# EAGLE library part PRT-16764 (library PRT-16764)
Headers & Wire Housings Extended GPIO Female Header - 2x20 Pin (13.5mm/9.80mm) Source: Datasheet
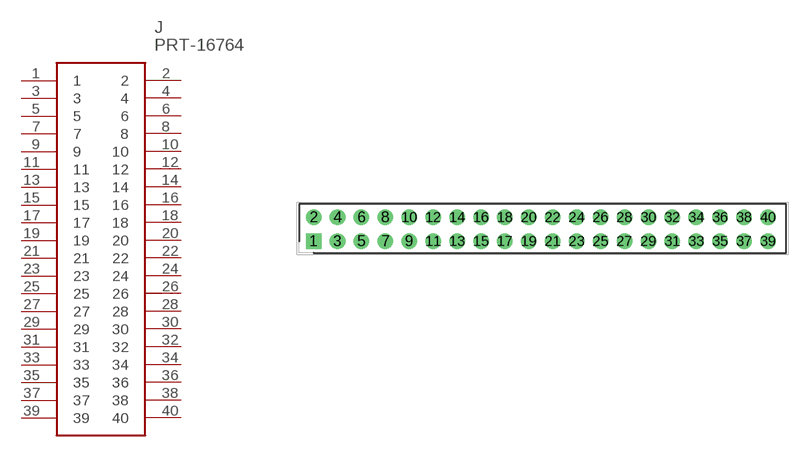
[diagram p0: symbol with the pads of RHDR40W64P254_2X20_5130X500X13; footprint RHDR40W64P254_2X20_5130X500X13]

Designator prefix J

## PRT-16764 (Description: Headers & Wire Housings Extended GPIO Female Header - 2x20 Pin (13.5mm/9.80mm); Height: 13.75mm; Manufacturer_Name: SparkFun; Manufacturer_Part_Number: PRT-16764; Mouser_Part_Number: 474-PRT-16764; Mouser_Price-Stock: https://www.mouser.co.uk/ProductDetail/SparkFun/PRT-16764?qs=W%2FMpXkg%252BdQ4FKwyaXnhaEw%3D%3D)  [RHDR40W64P254_2X20_5130X500X13]
1  1
2  2
3  3
4  4
5  5
6  6
7  7
8  8
9  9
10  10
11  11
12  12
13  13
14  14
15  15
16  16
17  17
18  18
19  19
20  20
21  21
22  22
23  23
24  24
25  25
26  26
27  27
28  28
29  29
30  30
31  31
32  32
33  33
34  34
35  35
36  36
37  37
38  38
39  39
40  40

## Footprint RHDR40W64P254_2X20_5130X500X13 (pad centres in mm)
PRT-16764
drill 1.1 pad 1.65 square: 1 0,0
drill 1.1 pad 1.65: 2 0,2.54; 3 2.54,0; 4 2.54,2.54; 5 5.08,0; 6 5.08,2.54; 7 7.62,0; 8 7.62,2.54; 9 10.16,0; 10 10.16,2.54; 11 12.7,0; 12 12.7,2.54; 13 15.24,0; 14 15.24,2.54; 15 17.78,0; 16 17.78,2.54; 17 20.32,0; 18 20.32,2.54; 19 22.86,0; 20 22.86,2.54; 21 25.4,0; 22 25.4,2.54; 23 27.94,0; 24 27.94,2.54; 25 30.48,0; 26 30.48,2.54; 27 33.02,0; 28 33.02,2.54; 29 35.56,0; 30 35.56,2.54; 31 38.1,0; 32 38.1,2.54; 33 40.64,0; 34 40.64,2.54; 35 43.18,0; 36 43.18,2.54; 37 45.72,0; 38 45.72,2.54; 39 48.26,0; 40 48.26,2.54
